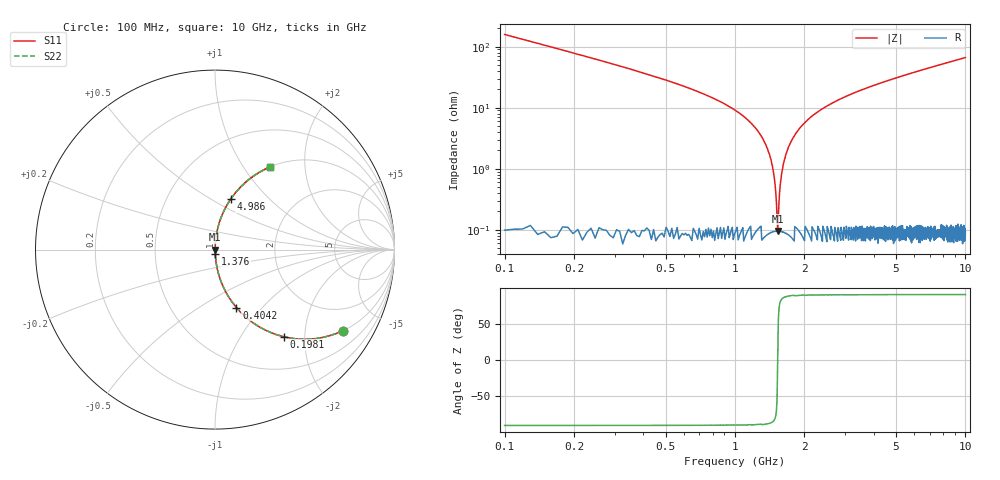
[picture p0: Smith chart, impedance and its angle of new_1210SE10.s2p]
!	AVX	Thin	Film	Operation	Date:	April 2007
!	Description:	Accu-P®	"Series,"	Thin	"Film,"	"SMD,"	RF	Capacitor
!	Part	Number:	12101J100FBT
!	100	MHz	-	5.05	GHz
!	Serial	Measurements
#	MHZ	S	MA	R	50
!	S11	S21	S12	S22
!	dB	Phase	dB	Phase	dB	Phase	dB	Phase
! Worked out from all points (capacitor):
!   1010 points, 100 MHz to 10 GHz, reference 50 ohm
!   read as one part in series: C = 10 pF near 149.1 MHz
!   lowest |Z| = 95.3 mohm at 1.533 GHz (marker M1)
!   series resonance near 1.532 GHz, so ESL is about 1.1 nH
!   S11 on the Smith chart (normalised r, x): 100 MHz: 1.00, -3.17; 198.1 MHz: 1.00, -1.58; 404.2 MHz: 1.00, -0.73; 1.376 GHz: 1.00, -0.04; 4.986 GHz: 1.00, +0.61; 10 GHz: 1.00, +1.32
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100  0.845 -32.2  0.534 57.7  0.534 57.7  0.845 -32.2
198.117  0.62 -51.7  0.784 38.3  0.784 38.3  0.62 -51.7
286.422  0.472 -61.7  0.881 28.2  0.881 28.2  0.472 -61.7
404.163  0.344 -69.8  0.938 20.1  0.938 20.1  0.344 -69.8
1090.981  0.072 -85.2  0.997 4.1  0.997 4.1  0.072 -85.2
1267.592  0.04 -86.4  0.998 2.3  0.998 2.3  0.04 -86.4
1375.52  0.022 -86.4  0.999 1.3  0.999 1.3  0.022 -86.4
1444.202  0.012 -85.1  0.999 0.7  0.999 0.7  0.012 -85.1
1503.072  0.00406 -77.0  0.999 0.2  0.999 0.2  0.00406 -77.0
1532.507  0.000902 4.2  0.999 -0.0  0.999 -0.0  0.000902 4.2
1561.943  0.00412 77.1  0.999 -0.2  0.999 -0.2  0.00412 77.1
1611.001  0.01 84.5  0.999 -0.6  0.999 -0.6  0.01 84.5
1640.436  0.014 85.6  0.999 -0.8  0.999 -0.8  0.014 85.6
1758.176  0.029 86.6  0.999 -1.6  0.999 -1.6  0.029 86.6
1964.222  0.052 86.0  0.998 -3.0  0.998 -3.0  0.052 86.0
2346.878  0.091 84.2  0.995 -5.2  0.995 -5.2  0.091 84.2
3406.541  0.181 79.3  0.983 -10.4  0.983 -10.4  0.181 79.3
4986.224  0.293 72.8  0.955 -17.0  0.955 -17.0  0.293 72.8
5054.906  0.297 72.6  0.954 -17.3  0.954 -17.3  0.297 72.6
6703.271  0.395 66.6  0.918 -23.3  0.918 -23.3  0.395 66.6
8351.635  0.48 61.2  0.877 -28.7  0.877 -28.7  0.48 61.2
10000  0.552 56.4  0.833 -33.5  0.833 -33.5  0.552 56.4
